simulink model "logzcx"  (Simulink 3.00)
settings: Solver=VariableStepDiscrete  SolverMode=SingleTasking  StartTime=0.0  StopTime=100  RelTol=1e-3  AbsTol=1e-6
libraries: simulink_extras x4

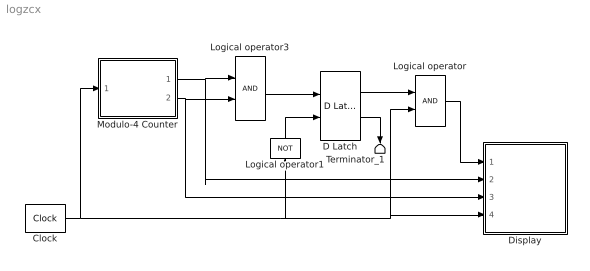
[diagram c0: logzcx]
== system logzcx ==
  Clock : simulink_extras/Flip Flops/Clock
  D Latch : simulink_extras/Flip Flops/D Latch
  Display : Subsystem
  Logical operator : Logic  Operator=AND  Inputs=2
  Logical operator1 : Logic  Orientation=up  Operator=NOT  Inputs=1
  Logical operator3 : Logic  Operator=AND  Inputs=2
  Modulo-4 Counter : Subsystem
  Terminator_1 : Terminator
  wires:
  Logical operator3/1 -> D Latch/1
  Logical operator1/1 -> D Latch/2
  D Latch/1 -> Logical operator/1
  Logical operator/1 -> Display/1(Output Pulse)
  Modulo-4 Counter/2(Low-Order Bit) -> Logical operator3/2, Display/3(Counter LSB)
  Clock/1 -> Logical operator1/1, Display/4(Clock), Logical operator/2, Modulo-4 Counter/1(Clock)
  Modulo-4 Counter/1(High-Order Bit) -> Logical operator3/1, Display/2(Counter MSB)
  D Latch/2 -> Terminator_1/1

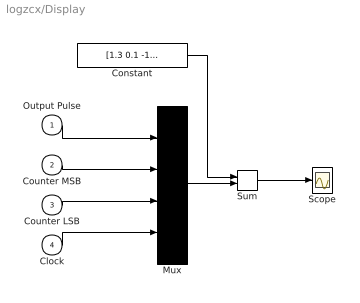
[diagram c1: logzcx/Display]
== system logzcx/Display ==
  Output Pulse : Inport  Port=1  PortWidth=-1  SampleTime=-1  DataType=auto
  Counter MSB : Inport  Port=2  PortWidth=-1  SampleTime=-1  DataType=auto
  Counter LSB : Inport  Port=3  PortWidth=-1  SampleTime=-1  DataType=auto
  Clock : Inport  Port=4  PortWidth=-1  SampleTime=-1  DataType=auto
  Constant : Constant  Value=[1.3 0.1 -1.2 -2.4]
  Mux : Mux  Inputs=4
  Scope : Scope
  Sum : Sum  Inputs=++  SaturateOnIntegerOverflow=on
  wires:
  Sum/1 -> Scope/1
  Counter MSB/1 -> Mux/2
  Counter LSB/1 -> Mux/3
  Clock/1 -> Mux/4
  Constant/1 -> Sum/1
  Mux/1 -> Sum/2
  Output Pulse/1 -> Mux/1

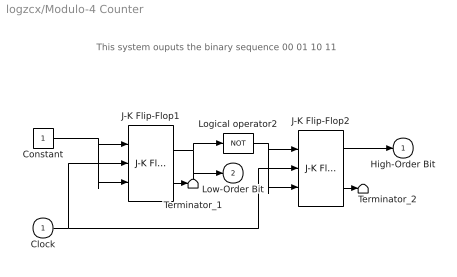
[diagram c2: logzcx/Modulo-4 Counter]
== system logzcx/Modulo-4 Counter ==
  note: This system ouputs the binary sequence 00 01 10 11
  Clock : Inport  Port=1  PortWidth=-1  SampleTime=-1  DataType=auto
  Constant : Constant  Value=1
  J-K Flip-Flop1 : simulink_extras/Flip Flops/J-K Flip-Flop  initial_condition=0
  J-K Flip-Flop2 : simulink_extras/Flip Flops/J-K Flip-Flop  initial_condition=0
  Logical operator2 : Logic  Operator=NOT  Inputs=1
  Terminator_1 : Terminator
  Terminator_2 : Terminator
  High-Order Bit : Outport  Port=1  InitialOutput=0
  Low-Order Bit : Outport  Port=2  InitialOutput=0
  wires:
  J-K Flip-Flop2/2 -> Terminator_2/1
  J-K Flip-Flop1/2 -> Terminator_1/1
  Logical operator2/1 -> J-K Flip-Flop2/3, J-K Flip-Flop2/1
  J-K Flip-Flop1/1 -> Logical operator2/1, Low-Order Bit/1
  Constant/1 -> J-K Flip-Flop1/1, J-K Flip-Flop1/3
  Clock/1 -> J-K Flip-Flop1/2, J-K Flip-Flop2/2
  J-K Flip-Flop2/1 -> High-Order Bit/1
